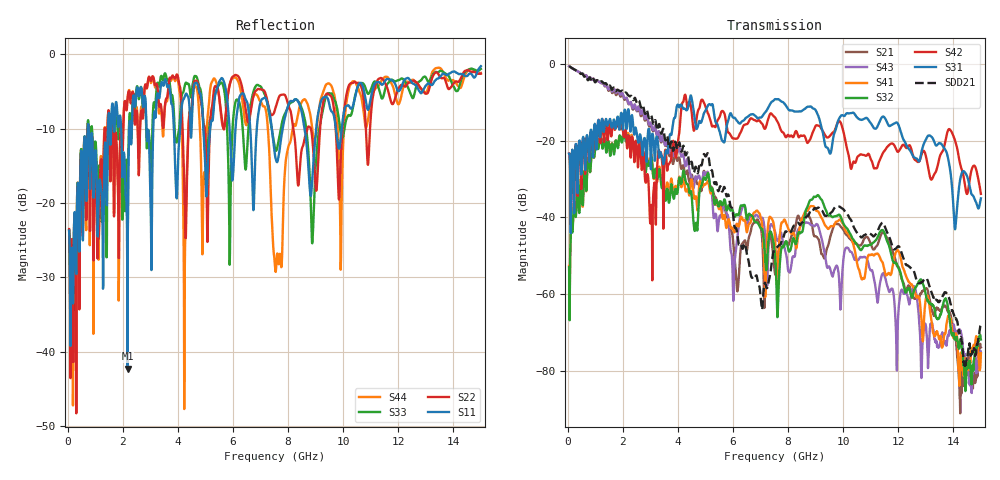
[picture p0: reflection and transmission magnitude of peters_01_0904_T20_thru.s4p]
# MHZ S RI R 50.00
! FREQ  S11  S12  S13  S14
!  S21  S22  S23  S24
!  S31  S32  S33  S34
!  S41  S42  S43  S44
!  REAL  IMAG  REAL  IMAG  REAL  IMAG  REAL  IMAG
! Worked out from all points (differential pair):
!   1496 points, 50 MHz to 15 GHz, reference 50 ohm
!   strongest paths, dB at 50 MHz, 3.79 GHz, 7.53 GHz, 11.27 GHz, 15 GHz:
!     S31: -23.4, -17.3, -9.2, -15.9, -35.0
!     S42: -23.4, -21.7, -14.0, -26.2, -33.9
!     S32: -53.1, -32.5, -50.1, -44.9, -71.8
!     S41: -52.7, -31.1, -45.8, -49.5, -75.4
!     S43: -0.6, -23.1, -43.8, -61.3, -75.2
!     S21: -0.6, -24.9, -54.9, -46.7, -73.9
!   taken as a pair (ports 3,1 in; 4,2 out), SDD21 dB: -0.6, -21.4, -48.3, -43.3, -67.9
!   lowest |S11| = -42.3 dB at 2.17 GHz (marker M1), VSWR 1.02, Z = 50.8 - j0.124 ohm
!   |S11| at or under -10 dB: start of sweep to 726.5 MHz; 761.4 MHz to 1.459 GHz (697.6 MHz wide, 62.8 % of centre); 8.593 GHz to 9.021 GHz (427.3 MHz wide, 4.85 % of centre)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
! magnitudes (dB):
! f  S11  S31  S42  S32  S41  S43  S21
! 50 MHz  -23.7  -23.4  -23.4  -53.1  -52.7  -0.6  -0.6
! 2.17 GHz  -42.3  -13.5  -21.5  -18.7  -18.2  -9.4  -9.7
! 3.03 GHz  -25.6  -25.7  -36.7  -24.2  -23.6  -15.6  -16.2
! 6.16 GHz  -7.5  -14.9  -19.4  -39.4  -41.8  -45.0  -59.3
! 7.59 GHz  -14.5  -9.2  -14.8  -60.6  -57.1  -45.8  -52.4
! 9.08 GHz  -8.2  -13.3  -16.1  -34.2  -38.4  -42.0  -45.4
! 15 GHz  -1.6  -35.0  -33.9  -71.8  -75.4  -75.2  -73.9
